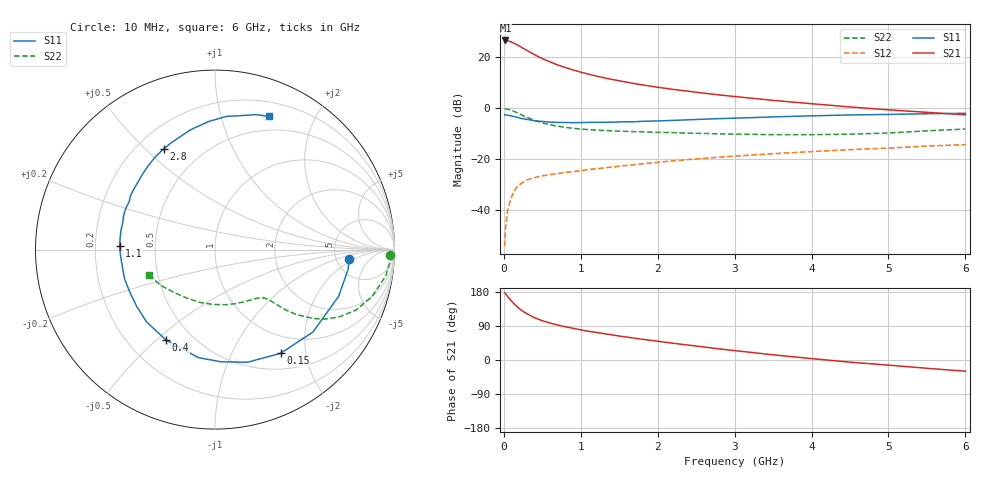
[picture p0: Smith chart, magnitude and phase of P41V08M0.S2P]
! SIEMENS Small Signal Semiconductors
! BFP182
! Si NPN RF Bipolar Junction Transistor in SOT143
! VCE = 1 V  IC = 8 mA
! Common Emitter S-Parameters:  March  1996
# GHz  S  MA  R  50
!  f  S11  S21  S12  S22
! GHz  MAG  ANG  MAG  ANG  MAG  ANG  MAG  ANG
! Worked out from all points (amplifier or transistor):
!   36 points, 10 MHz to 6 GHz, reference 50 ohm
!   highest |S21| = 26.6 dB at 20 MHz (marker M1)
!   |S21| within 3 dB of that: start of sweep to 246.4 MHz
!   unconditionally stable (mu >= 1): 1.133 GHz to end of sweep
!   at 250 MHz: K = 0.32, MSG = 26.2 dB, |S12| = -28.9 dB
!   at 1.4 GHz: K = 1.11, MAG = 15.1 dB, |S12| = -23.0 dB
!   at 6 GHz: K = 1.02, MAG = 5.0 dB, |S12| = -14.2 dB
!   S11 on the Smith chart (normalised r, x): 10 MHz: 6.54, -1.63; 150 MHz: 0.72, -1.57; 400 MHz: 0.36, -0.54; 1.1 GHz: 0.31, +0.02; 2.8 GHz: 0.31, +0.57; 6 GHz: 0.34, +1.43
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0.01  0.7486 -4.2  21.3 177.6  0.002 86.0  0.9778 -1.7
0.02  0.7496 -8.4  21.43 175.3  0.0042 82.6  0.9789 -3.5
0.05  0.7364 -20.7  21.12 167.3  0.0103 82.1  0.9629 -8.7
0.1  0.7132 -40.1  19.84 155.4  0.0186 70.7  0.913 -16.7
0.15  0.6837 -57.7  18.32 144.8  0.0264 62.6  0.8534 -23.3
0.2  0.6532 -73.9  16.77 135.7  0.0319 57.5  0.7865 -28.5
0.25  0.626 -86.9  15.05 128.1  0.0357 51.8  0.7229 -32.4
0.3  0.6091 -98.7  13.65 122.1  0.0397 48.4  0.6693 -35.0
0.4  0.5726 -118.4  11.28 111.4  0.0441 43.3  0.5821 -38.5
0.5  0.555 -133.3  9.443 103.7  0.0477 40.7  0.5199 -40.4
0.6  0.5392 -143.9  8.167 97.6  0.0506 39.2  0.4782 -41.3
0.7  0.5304 -153.8  7.074 92.2  0.0529 38.8  0.449 -42.0
0.9  0.5251 -169.2  5.675 83.6  0.0577 38.4  0.4074 -43.0
1.1  0.5322 177.9  4.695 75.8  0.0633 38.6  0.3844 -44.7
1.5  0.5431 159.7  3.471 63.2  0.0737 39.1  0.3594 -48.9
1.8  0.5581 147.6  2.893 54.7  0.0821 39.3  0.3474 -53.3
2.2  0.5818 134.3  2.358 44.2  0.0938 38.0  0.3353 -60.4
2.8  0.6295 117.0  1.836 29.3  0.1109 35.0  0.3167 -73.3
3.5  0.6809 101.7  1.436 13.7  0.1293 30.4  0.3059 -91.5
4.5  0.7448 85.1  1.068 -5.7  0.1553 23.3  0.3126 -120.4
5.5  0.7853 73.3  0.838 -21.9  0.1834 16.1  0.3637 -147.0
6  0.8014 67.9  0.749 -29.6  0.1948 11.4  0.3942 -159.3
